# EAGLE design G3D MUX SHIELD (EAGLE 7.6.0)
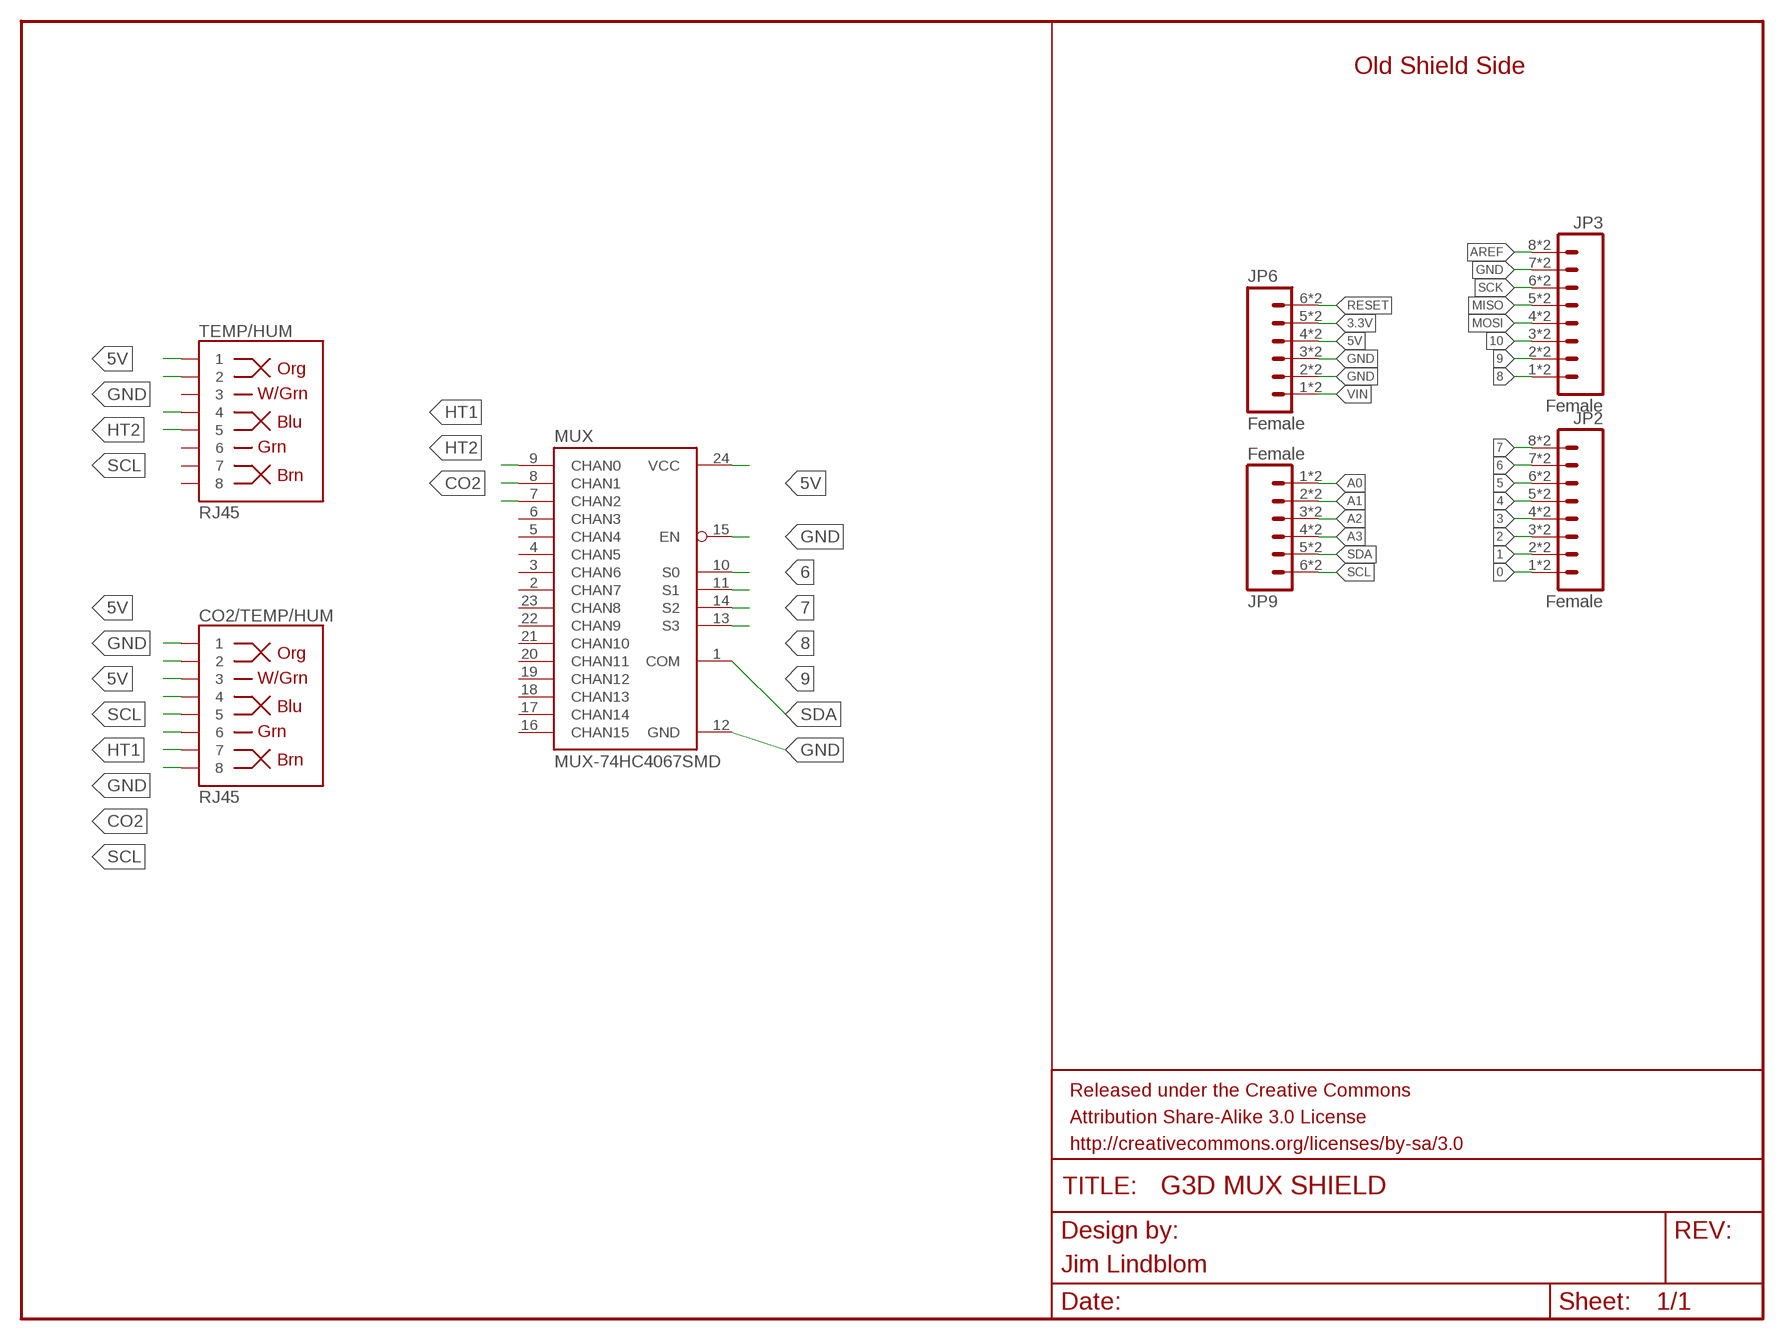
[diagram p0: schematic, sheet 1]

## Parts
CO2/TEMP/HUM  RJ45  RJ45-8PTH  [RJ45-8]
JP2  Female  M08SMD-COMBO  [1X08_SMD_COMBINED]
JP3  Female  M08SMD-COMBO  [1X08_SMD_COMBINED]
JP6  Female  M06SMD-STRAIGHT-COMBO  [1X06_SMD_STRAIGHT_COMBO]
JP9  Female  M06SMD-STRAIGHT-COMBO  [1X06_SMD_STRAIGHT_COMBO]
MUX  MUX-74HC4067SMD  [SSOP24]
TEMP/HUM  RJ45  RJ45-8PTH  [RJ45-8]

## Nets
0: JP2.1 JP2.1@2
1: JP2.2 JP2.2@2
2: JP2.3 JP2.3@2
3: JP2.4 JP2.4@2
3.3V: JP6.5 JP6.5-2
4: JP2.5 JP2.5@2
5: JP2.6 JP2.6@2
5V: CO2/TEMP/HUM.1 CO2/TEMP/HUM.3 JP6.4 JP6.4-2 MUX.24(VCC) TEMP/HUM.1
6: JP2.7 JP2.7@2 MUX.10(S0)
7: JP2.8 JP2.8@2 MUX.11(S1)
8: JP3.1 JP3.1@2 MUX.14(S2)
9: JP3.2 JP3.2@2 MUX.13(S3)
10: JP3.3 JP3.3@2
A0: JP9.1 JP9.1-2
A1: JP9.2 JP9.2-2
A2: JP9.3 JP9.3-2
A3: JP9.4 JP9.4-2
AREF: JP3.8 JP3.8@2
CO2: CO2/TEMP/HUM.7 MUX.7(CHAN2)
GND: CO2/TEMP/HUM.2 CO2/TEMP/HUM.6 JP3.7 JP3.7@2 JP6.2 JP6.2-2 JP6.3 JP6.3-2 MUX.12(GND) MUX.15(EN) TEMP/HUM.2
HT1: CO2/TEMP/HUM.5 MUX.9(CHAN0)
HT2: MUX.8(CHAN1) TEMP/HUM.4
MISO: JP3.5 JP3.5@2
MOSI: JP3.4 JP3.4@2
RESET: JP6.6 JP6.6-2
SCK: JP3.6 JP3.6@2
SCL: CO2/TEMP/HUM.4 CO2/TEMP/HUM.8 JP9.6 JP9.6-2 TEMP/HUM.5
SDA: JP9.5 JP9.5-2 MUX.1(COM)
VIN: JP6.1 JP6.1-2
Unconnected: MUX.2(CHAN7) MUX.3(CHAN6) MUX.4(CHAN5) MUX.5(CHAN4) MUX.6(CHAN3) MUX.16(CHAN15) MUX.17(CHAN14) MUX.18(CHAN13) MUX.19(CHAN12) MUX.20(CHAN11) MUX.21(CHAN10) MUX.22(CHAN9) MUX.23(CHAN8) TEMP/HUM.3 TEMP/HUM.6 TEMP/HUM.7 TEMP/HUM.8

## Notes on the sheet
- Old Shield Side
- Jim Lindblom

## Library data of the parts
CO2/TEMP/HUM TEMP/HUM = SparkFun-Connectors:RJ45-8: RJ45 Jack Simple RJ45, 8-pin connection - connector for common Cat5, Cat5e, and Cat6 Ethernet cables. Footprint not yet proven in production. Connector sku is PRT-00643; Breakout PCB sku is BOB-00716.; PROD_ID: CONN-08506
JP2 JP3 = SparkFun-Connectors:M08: Header 8 Standard 8-pin 0.1" header. Use with straight break away headers (SKU : PRT-00116), right angle break away headers (PRT-00553), swiss pins (PRT-00743), machine pins (PRT-00117), and female headers (PRT-00115).
JP6 JP9 = SparkFun-Connectors:M06: Header 6 Standard 6-pin 0.1" header. Use with straight break away headers (SKU : PRT-00116), right angle break away headers (PRT-00553), swiss pins (PRT-00743), machine pins (PRT-00117), and female headers (PRT-00115). Molex polarized connector foot print use with SKU : PRT-08094 with associated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
MUX = SparkFun-AnalogIC:MUX-74HC4067: 16-channel analog MUX; PROD_ID: IC-08252

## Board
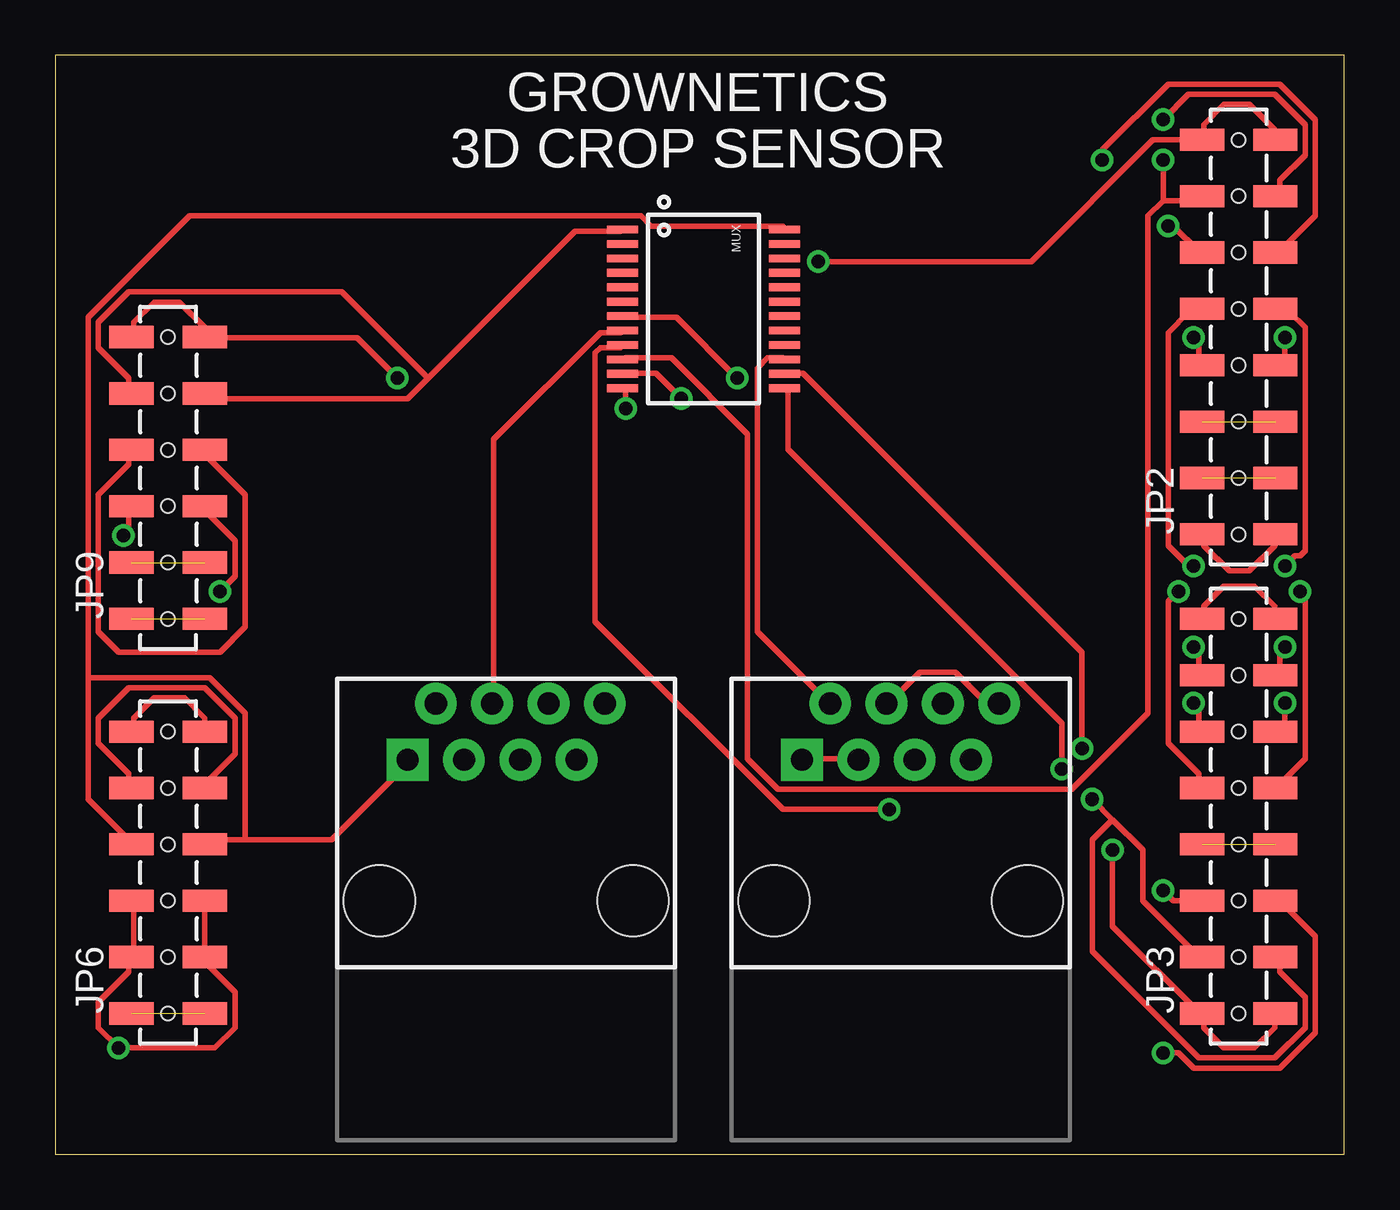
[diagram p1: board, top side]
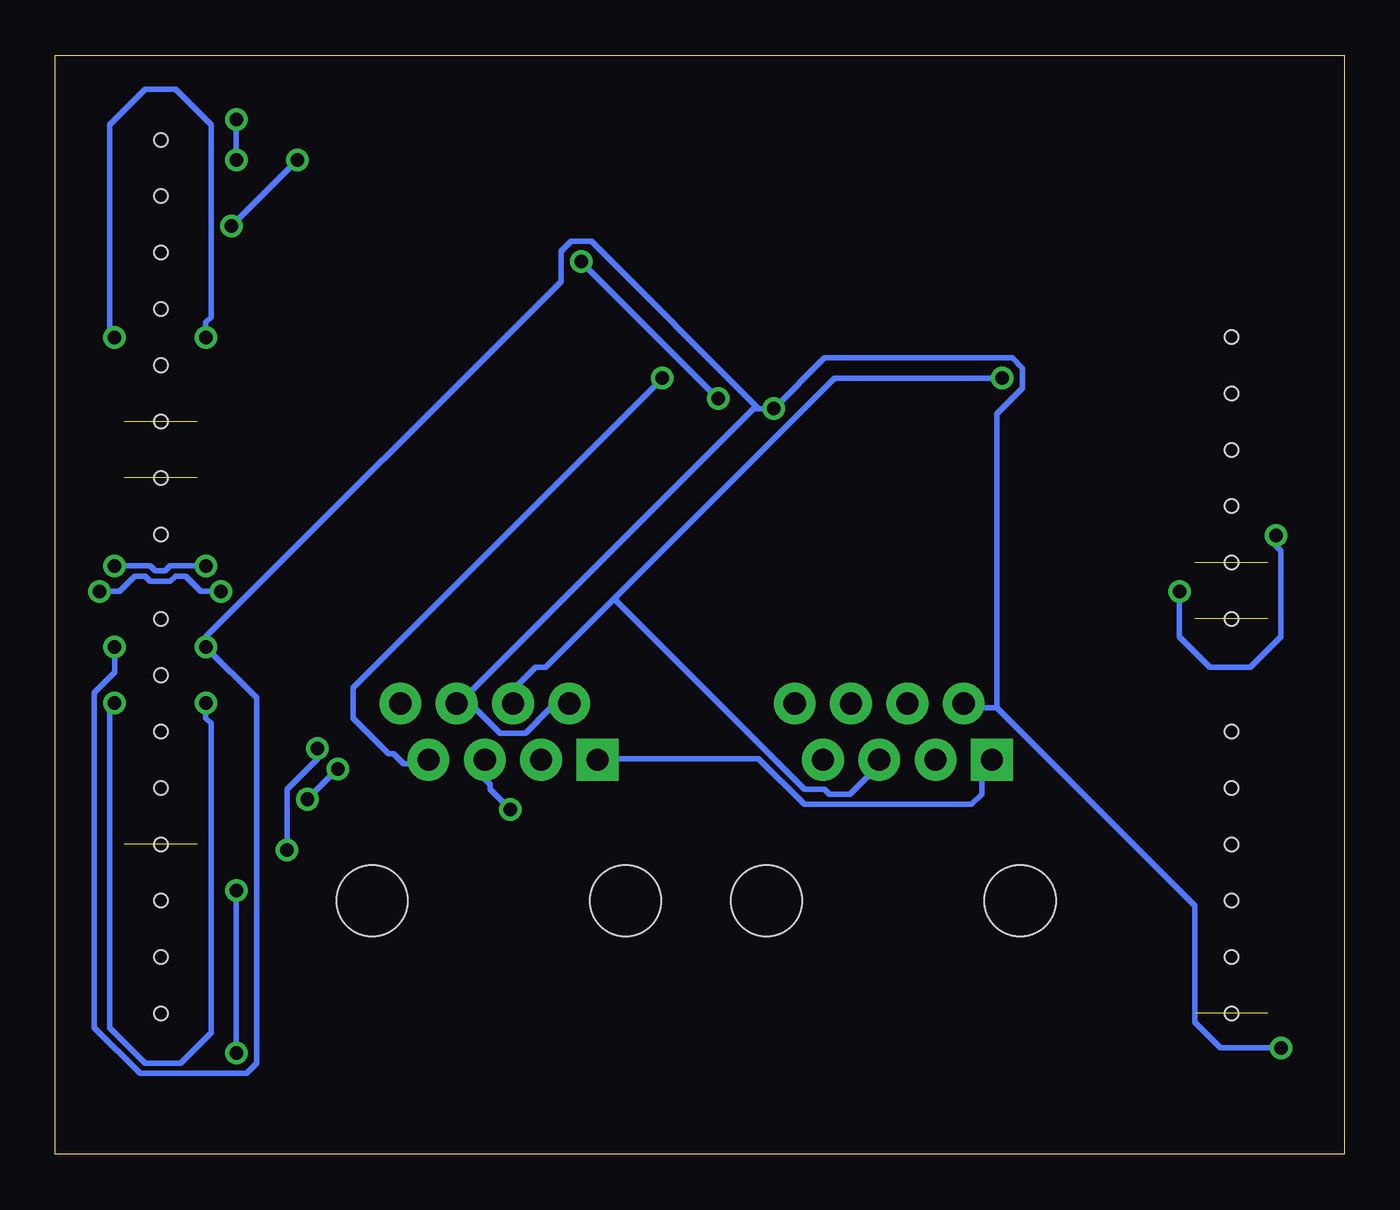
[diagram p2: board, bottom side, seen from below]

Size 58.09 x 49.52 mm. Coordinates in mm from the lower left corner, seen from the top.
Outline: 0,0 58.09,0 58.09,49.52 0,49.52 0,0
Copper layers (1*16): Top 0.035mm / dielectric 1.5mm / Bottom 0.035mm
Design rules "default": minimum track width 10mil, minimum drill 24mil, track to track 8mil, track to pad 8mil, pad to pad 8mil, via to via 8mil, smd to smd 8mil, copper to edge 40mil, drill to drill 8mil, minimum pad ring 10mil, minimum via ring 8mil, stop-mask expansion 4mil, vias tented up to drill 0mil, thermal gap 10mil
Holes 0.6 mm at 5.08,36.83 5.08,34.29 5.08,31.75 5.08,29.21 5.08,26.67 5.08,24.13 5.08,19.05 5.08,16.51 5.08,13.97 5.08,11.43 5.08,8.89 5.08,6.35 53.34,6.35 53.34,8.89 53.34,11.43 53.34,13.97 53.34,16.51 53.34,19.05 53.34,21.59 53.34,24.13 53.34,27.94 53.34,30.48 53.34,33.02 53.34,35.56 53.34,38.1 53.34,40.64 53.34,43.18 53.34,45.72

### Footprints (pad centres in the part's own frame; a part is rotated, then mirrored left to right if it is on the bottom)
RJ45-8 = drill 1 pad 1.88 square: 1 -4.445,6.35 | drill 1 pad 1.88: 2 -3.175,8.89; 3 -1.905,6.35; 4 -0.635,8.89; 5 0.635,6.35; 6 1.905,8.89; 7 3.175,6.35; 8 4.445,8.89 | hole 3.2: -5.715,0; 5.715,0
1X08_SMD_COMBINED = smd 1 x 2: 1 0,1.65; 1@2 0,-1.65; 2 2.54,-1.65; 2@2 2.54,1.65; 3 5.08,1.65; 3@2 5.08,-1.65; 4 7.62,-1.65; 4@2 7.62,1.65; 5 10.16,1.65; 5@2 10.16,-1.65; 6 12.7,-1.65; 6@2 12.7,1.65; 7 15.24,1.65; 7@2 15.24,-1.65; 8 17.78,-1.65; 8@2 17.78,1.65
1X06_SMD_STRAIGHT_COMBO = smd 1 x 2: 1 0,-1.65; 1-2 0,1.65; 2 2.54,1.65; 2-2 2.54,-1.65; 3 5.08,-1.65; 3-2 5.08,1.65; 4 7.62,1.65; 4-2 7.62,-1.65; 5 10.16,-1.65; 5-2 10.16,1.65; 6 12.7,1.65; 6-2 12.7,-1.65
SSOP24 = smd 0.348 x 1.397: 1 -3.575,-3.656; 2 -2.925,-3.656; 3 -2.275,-3.656; 4 -1.625,-3.656; 5 -0.975,-3.656; 6 -0.325,-3.656; 7 0.325,-3.656; 8 0.975,-3.656; 9 1.625,-3.656; 10 2.275,-3.656; 11 2.925,-3.656; 12 3.575,-3.656; 13 3.575,3.656; 14 2.925,3.656; 15 2.275,3.656; 16 1.625,3.656; 17 0.975,3.656; 18 0.325,3.656; 19 -0.325,3.656; 20 -0.975,3.656; 21 -1.625,3.656; 22 -2.275,3.656; 23 -2.925,3.656; 24 -3.575,3.656

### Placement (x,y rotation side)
CO2/TEMP/HUM  38.1,11.43 0 top
JP2  53.34,27.94 90 top
JP3  53.34,6.35 90 top
JP6  5.08,6.35 90 top
JP9  5.08,24.13 90 top
MUX  29.21,38.1 270 top
TEMP/HUM  20.32,11.43 0 top

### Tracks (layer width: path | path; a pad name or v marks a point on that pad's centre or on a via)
0
  Top 0.254: JP2.1 51.77,27.89 51.77,27.43 52.91,26.29 53.82,26.29 54.97,27.43 54.97,27.89 JP2.1@2
1  (1 unrouted)
2  (1 unrouted)
3  (via drill 0.61)
  Top 0.254: v51.31,36.8 51.54,36.58 51.54,35.66 JP2.4@2 | v55.42,36.8 55.42,35.89 55.19,35.66 JP2.4
  Bottom 0.254: v51.31,36.8 51.31,37.49 51.08,37.72 51.08,46.41 52.68,48.01 54.05,48.01 55.65,46.41 55.65,37.03 v55.42,36.8
3.3V
  Top 0.254: JP6.5-2 3.3,16.69 3.3,17.14 1.93,18.52 1.93,19.66 3.3,21.03 6.73,21.03 8.1,19.66 8.1,18.06 6.73,16.69 JP6.5
4  (via drill 0.61)
  Top 0.254: v51.31,26.52 51.08,26.52 50.17,27.43 50.17,37.03 51.08,37.95 51.54,37.95 JP2.5 | v55.42,26.52 55.88,26.98 56.11,26.98 56.34,27.2 56.34,37.26 55.65,37.95 55.19,37.95 JP2.5@2
  Bottom 0.254: v51.31,26.52 52.91,26.52 53.14,26.29 53.59,26.29 53.82,26.52 v55.42,26.52
5  (via drill 0.61)
  Top 0.254: v50.17,41.83 50.39,41.83 51.54,40.69 JP2.6@2 | v47.19,44.81 47.19,45.26 50.17,48.23 55.19,48.23 56.79,46.63 56.79,42.29 55.19,40.69 JP2.6
  Bottom 0.254: v47.19,44.81 v50.17,41.83
5V
  Top 0.254: CO2/TEMP/HUM.1 33.71,17.83 35.99,17.83 CO2/TEMP/HUM.3 | 8.56,14.17 12.45,14.17 15.88,17.6 TEMP/HUM.1 | 8.56,14.17 6.73,14.17 JP6.4-2 | 1.47,21.49 1.47,16 3.3,14.17 JP6.4 | 1.47,21.49 1.47,37.72 6.05,42.29 26.39,42.29 26.85,41.83 32.79,41.83 MUX.24 | 8.56,14.17 8.56,19.89 6.96,21.49 1.47,21.49
  Bottom 0.254: CO2/TEMP/HUM.1 33.48,17.83 26.39,17.83 24.33,15.77 16.79,15.77 16.33,16.23 16.33,17.14 15.88,17.6 TEMP/HUM.1
6  (via drill 0.61)
  Top 0.254: 49.94,42.98 49.25,42.29 49.25,19.89 45.82,16.46 32.56,16.46 31.19,17.83 31.19,32.46 27.76,35.89 25.71,35.89 MUX.10 | 49.94,42.98 51.54,42.98 JP2.7 | v49.94,46.63 51.08,47.78 54.97,47.78 56.34,46.41 56.34,45.03 55.19,43.89 55.19,43.2 JP2.7@2 | 49.94,42.98 v49.94,44.81
  Bottom 0.254: v49.94,44.81 v49.94,46.63
7  (via drill 0.61)
  Top 0.254: v28.22,34.06 27.08,35.2 25.71,35.2 MUX.11 | v34.39,40.23 43.99,40.23 49.48,45.72 JP2.8@2 51.77,45.72 51.77,46.41 52.68,47.32 53.82,47.32 54.97,46.18 54.97,45.72 JP2.8
  Bottom 0.254: v34.39,40.23 v28.22,34.06
8  (via drill 0.61)
  Top 0.254: v46.28,18.29 46.28,22.63 33.71,35.2 33.02,35.2 MUX.14 | v47.65,13.72 47.65,10.29 51.54,6.4 JP3.1 51.77,6.17 51.77,5.71 52.68,4.8 54.05,4.8 54.97,5.71 54.97,6.17 JP3.1@2
  Bottom 0.254: v46.28,18.29 46.28,17.83 47.65,16.46 v47.65,13.72
9  (via drill 0.61)
  Top 0.254: v45.36,17.37 45.36,19.43 33.02,31.77 33.02,34.52 MUX.13 | 47.65,15.09 49.02,13.72 49.02,11.43 51.54,8.91 JP3.2@2 | 47.65,15.09 v46.74,16 | 47.65,15.09 46.74,14.17 46.74,9.14 51.54,4.34 54.97,4.34 56.34,5.71 56.34,7.09 55.19,8.23 55.19,8.69 JP3.2
  Bottom 0.254: v46.74,16 v45.36,17.37
10  (via drill 0.61)
  Top 0.254: JP3.3 50.39,11.43 v49.94,11.89 | v49.94,4.57 50.62,4.57 51.31,3.89 55.19,3.89 56.79,5.49 56.79,9.83 55.19,11.43 JP3.3@2
  Bottom 0.254: v49.94,4.57 v49.94,11.89
A0  (1 unrouted)
A1  (1 unrouted)
A2  (via drill 0.61)
  Top 0.254: v3.07,27.89 3.3,28.12 3.3,29.03 JP9.3-2 | v7.42,25.38 8.1,26.06 8.1,27.66 6.73,29.03 JP9.3
  Bottom 0.254: v3.07,27.89 3.07,27.43 2.85,27.2 2.85,23.32 4.22,21.95 6.05,21.95 7.42,23.32 v7.42,25.38
A3
  Top 0.254: JP9.4 3.3,31.55 3.3,31.09 1.93,29.72 1.93,23.55 2.85,22.63 7.42,22.63 8.56,23.77 8.56,29.72 6.73,31.55 JP9.4-2
AREF
  Top 0.254: JP3.8@2 51.77,24.23 51.77,24.69 52.68,25.6 54.05,25.6 54.97,24.69 54.97,24.23 JP3.8
CO2  (via drill 0.61)
  Top 0.254: v30.73,34.98 27.99,37.72 25.71,37.72 MUX.7
  Bottom 0.254: v30.73,34.98 44.68,21.03 44.68,19.66 43.08,18.06 42.85,18.06 42.39,17.6 41.48,17.6 CO2/TEMP/HUM.7
GND  (via drill 0.61)
  Top 0.254: JP6.3-2 3.53,11.43 3.53,8.91 JP6.2 3.3,8.69 3.3,8.23 1.93,6.86 1.93,5.71 v2.85,4.8 7.19,4.8 8.1,5.71 8.1,7.32 6.73,8.69 JP6.2-2 6.73,8.91 JP6.3 | v25.71,33.6 25.71,34.52 MUX.12 | MUX.15 32.79,35.89 32.11,35.89 31.65,35.43 31.65,23.55 34.85,20.34 CO2/TEMP/HUM.2 | v51.31,22.86 51.54,22.63 51.54,21.72 JP3.7 | v55.42,22.86 55.19,22.63 55.19,21.72 JP3.7@2
  Bottom 0.254: 15.65,20.12 17.02,20.12 TEMP/HUM.2 | 15.65,20.12 6.73,11.2 6.73,5.94 5.59,4.8 v2.85,4.8 | 26.39,33.6 26.62,33.6 39.65,20.57 | 26.39,33.6 v25.71,33.6 23.42,35.89 14.96,35.89 14.5,35.43 14.5,34.52 15.65,33.38 15.65,20.12 | 39.65,20.57 39.88,20.34 CO2/TEMP/HUM.6 39.65,20.57 | 26.39,33.6 33.93,41.15 34.85,41.15 35.31,40.69 35.31,39.32 51.31,23.32 v51.31,22.86 49.02,20.57 49.02,4.12 49.48,3.66 54.28,3.66 56.34,5.71 56.34,20.8 55.42,21.72 v55.42,22.86 | 39.65,20.57 38.05,18.97 36.91,18.97 35.76,20.12 35.08,20.12 CO2/TEMP/HUM.2
HT1  (via drill 0.61)
  Top 0.254: v37.59,15.55 32.79,15.55 24.33,24 24.33,36.12 24.56,36.35 25.48,36.35 MUX.9
  Bottom 0.254: v37.59,15.55 38.51,16.46 38.51,16.69 38.73,16.92 CO2/TEMP/HUM.5
HT2
  Top 0.254: MUX.8 25.48,37.03 24.56,37.03 19.76,32.23 19.76,20.34 TEMP/HUM.4
MISO  (via drill 0.61)
  Top 0.254: v50.62,25.38 50.17,24.92 50.17,18.52 51.54,17.14 51.54,16.69 JP3.5 | v56.11,25.38 56.11,25.15 56.34,24.92 56.34,17.83 55.19,16.69 JP3.5@2
  Bottom 0.254: v50.62,25.38 51.54,25.38 52.22,26.06 52.68,26.06 52.91,25.83 53.82,25.83 54.05,26.06 54.51,26.06 55.19,25.38 v56.11,25.38
MOSI  (1 unrouted)
RESET
  Top 0.254: JP6.6 3.53,19.2 3.53,19.66 4.45,20.57 5.82,20.57 6.73,19.66 6.73,19.2 JP6.6-2
SCK  (via drill 0.61)
  Top 0.254: v51.31,20.34 51.54,20.12 51.54,19.2 JP3.6@2 | v55.42,20.34 55.42,19.43 55.19,19.2 JP3.6
  Bottom 0.254: v51.31,20.34 51.31,19.66 51.08,19.43 51.08,5.49 52.45,4.12 54.05,4.12 55.65,5.71 55.65,20.12 v55.42,20.34
SCL  (via drill 0.61)
  Top 0.254: JP9.6 3.53,37.03 3.53,37.49 4.45,38.41 5.59,38.41 6.73,37.26 6.73,37.03 JP9.6-2 6.73,36.8 13.59,36.8 v15.42,34.98 | CO2/TEMP/HUM.8 42.39,20.34 41.94,20.34 40.56,21.72 38.96,21.72 37.59,20.34 CO2/TEMP/HUM.4
  Bottom 0.254: v15.42,34.98 22.96,34.98 32.79,25.15 | 32.79,25.15 35.99,21.95 36.45,21.95 37.36,21.03 37.36,20.34 CO2/TEMP/HUM.4 | 32.79,25.15 32.79,24.92 24.33,16.46 23.42,16.46 23.19,16.23 22.28,16.23 21.13,17.37 21.13,17.6 TEMP/HUM.5
SDA
  Top 0.254: 16.79,34.98 15.88,34.06 6.96,34.06 JP9.5 | 16.79,34.98 23.42,41.6 25.48,41.6 MUX.1 | 16.79,34.98 12.9,38.86 3.3,38.86 1.93,37.49 1.93,36.35 3.3,34.98 3.3,34.29 JP9.5-2
VIN  (1 unrouted)

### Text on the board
tPlace: GROWNETICS | 3D CROP SENSOR

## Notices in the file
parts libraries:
SparkFun-Aesthetics: Licensing: CC v3.0 Share-Alike You are welcome to use this library for commercial purposes.
SparkFun-Aesthetics: Released under the Creative Commons
SparkFun-Aesthetics: http://creativecommons.org/licenses/by-sa/3.0
